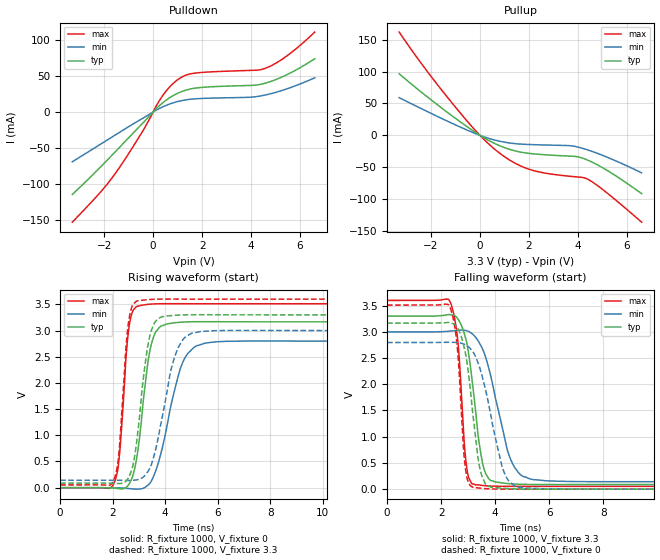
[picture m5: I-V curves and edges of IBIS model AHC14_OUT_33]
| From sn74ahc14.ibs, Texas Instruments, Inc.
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[Model]   AHC14_OUT_33
Model_type  Output
Vref =   0
Rref =   1000
Cref =   50p
Vmeas =   1.65
| variable   typ   min   max
C_comp   2.83pF   1.52pF   3.97pF
| C_pullup   2.81pF   1.52pF   3.53pF
| C_pulldown   2.86pF   1.73pF   3.97pF
[Temperature Range]   40   100   -40
| Ambient temperature   25   85   -40
[Voltage range]   3.3   3   3.6
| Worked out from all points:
|   slope of the pulldown table from 0 to 0.495 V, typ, clamps not added: 31.8 ohm
|   slope of the pullup table from 0 to 0.495 V, typ, clamps not added: 45.8 ohm
|   rising waveform, R_fixture 1000, V_fixture 0: 20-80 % time 449ps typ, 769ps min, 291ps max; typ from 0 V to 3.17 V
|   falling waveform, R_fixture 1000, V_fixture 3.3: 20-80 % time 458ps typ, 770ps min, 271ps max; typ from 3.3 V to 0.088 V
|   rising waveform, R_fixture 1000, V_fixture 3.3: 20-80 % time 447ps typ, 690ps min, 289ps max; typ from 0.088 V to 3.3 V
|   falling waveform, R_fixture 1000, V_fixture 0: 20-80 % time 434ps typ, 723ps min, 261ps max; typ from 3.17 V to 0 V
[Pulldown]
| AHC14_OUT_33
|   Voltage   I(typ)   I(min)   I(max)
-3.3V     -114.4mA   -69.04mA   -152.9mA
-2.22V    -78.8mA    -46.22mA   -113.9mA
-1.635V   -58.39mA   -33.79mA   -89.51mA
-480mV    -17.44mA   -9.793mA   -29.54mA
330mV     11.04mA    6.164mA    19.74mA
635mV     18.98mA    10.63mA    33.32mA
955mV     25.27mA    14.14mA    43.64mA
1.295V    29.94mA    16.67mA    50.63mA
1.685V    33.04mA    18.27mA    53.93mA
4.555V    39.87mA    23.49mA    60.41mA
5.45V     51.66mA    32.05mA    77.66mA
6.6V      73.99mA    47.56mA    111mA
[Pullup]
| AHC14_OUT_33
|   Voltage   I(typ)   I(min)   I(max)
-3.3V     96.43mA    59.11mA    161.8mA
-2.19V    61.53mA    38.04mA    102.2mA
-995mV    26.52mA    16.31mA    43.97mA
-15mV     367.5uA    219.4uA    603.7uA
745mV     -15.3mA    -8.685mA   -26.19mA
1.415V    -24.13mA   -12.91mA   -43.25mA
2.085V    -28.58mA   -14.44mA   -54.08mA
3.69V     -32.57mA   -16.26mA   -64.18mA
4.03V     -33.95mA   -18.66mA   -65.36mA
4.39V     -38.7mA    -22.73mA   -68.57mA
5.315V    -57.85mA   -36.24mA   -94.18mA
6.6V      -91.36mA   -58.68mA   -136.1mA
[Ramp]
| AHC14_OUT_33
| variable   typ   min   max
dV/dt_r   1.91/4.68E-10   1.70/7.93E-10   2.12/3.09E-10
dV/dt_f   1.95/4.83E-10   1.74/8.15E-10   2.14/2.85E-10
R_load = 1000
[Rising Waveform]
| AHC14_OUT_33
R_fixture =   1000
C_fixture =   0
L_fixture =   0
V_fixture =   0
V_fixture_min = 0
V_fixture_max = 0
|   Time   V(typ)   V(min)   V(max)
0s        923.7pV    1.562nV    526.1pV
2.055ns   -8.312mV   -820.6uV   89.19mV
2.25ns    -20.16mV   -3.477mV   579.8mV
2.655ns   94.12mV    -18.6mV    3.168V
2.94ns    637.5mV    -28.26mV   3.466V
3.26ns    2.057V     15.51mV    3.495V
3.79ns    3.066V     563.2mV    3.512V
4.65ns    3.162V     2.369V     3.512V
5.615ns   3.17V      2.767V     3.511V
50ns      3.167V     2.797V     3.511V
[Falling Waveform]
| AHC14_OUT_33
R_fixture =   1000
C_fixture =   0
L_fixture =   0
V_fixture =   3.3
V_fixture_min = 3
V_fixture_max = 3.6
|   Time   V(typ)   V(min)   V(max)
0s        3.3V       3V         3.6V
2.33ns    3.329V     3.015V     3.578V
2.63ns    3.242V     3.03V      2.775V
2.945ns   2.802V     3.022V     429.2mV
3.285ns   1.453V     2.892V     81.78mV
3.525ns   519.2mV    2.683V     70.73mV
3.77ns    194.1mV    2.299V     60.13mV
4.57ns    101.9mV    573.1mV    52.56mV
5.445ns   88.04mV    178.4mV    52.29mV
50ns      87.98mV    143.4mV    52.56mV
[Rising Waveform]
| AHC14_OUT_33
R_fixture =   1000
C_fixture =   0
L_fixture =   0
V_fixture =   3.3
V_fixture_min = 3
V_fixture_max = 3.6
|   Time   V(typ)   V(min)   V(max)
0s        87.98mV    143.4mV    52.56mV
2.05ns    84.23mV    142.6mV    156.9mV
2.24ns    80.64mV    141.4mV    673.5mV
2.595ns   183.4mV    137.6mV    3.122V
2.955ns   1.04V      154.1mV    3.568V
3.305ns   2.6V       281.7mV    3.589V
3.585ns   3.138V     626.2mV    3.598V
4.425ns   3.293V     2.586V     3.601V
5.36ns    3.303V     2.982V     3.6V
50ns      3.3V       3V         3.6V
[Falling Waveform]
| AHC14_OUT_33
R_fixture =   1000
C_fixture =   0
L_fixture =   0
V_fixture =   0
V_fixture_min = 0
V_fixture_max = 0
|   Time   V(typ)   V(min)   V(max)
0s        3.167V     2.797V     3.511V
2.32ns    3.176V     2.801V     3.48V
2.59ns    3.087V     2.796V     2.758V
2.9ns     2.591V     2.754V     398.4mV
3.22ns    1.241V     2.586V     29.31mV
3.415ns   450.7mV    2.337V     20.22mV
3.655ns   91.23mV    1.874V     9mV
4.27ns    17.05mV    408.2mV    560.3uV
4.86ns    3.212mV    34.21mV    -200.5uV
50ns      4.439nV    -36.08nV   -9.937nV
